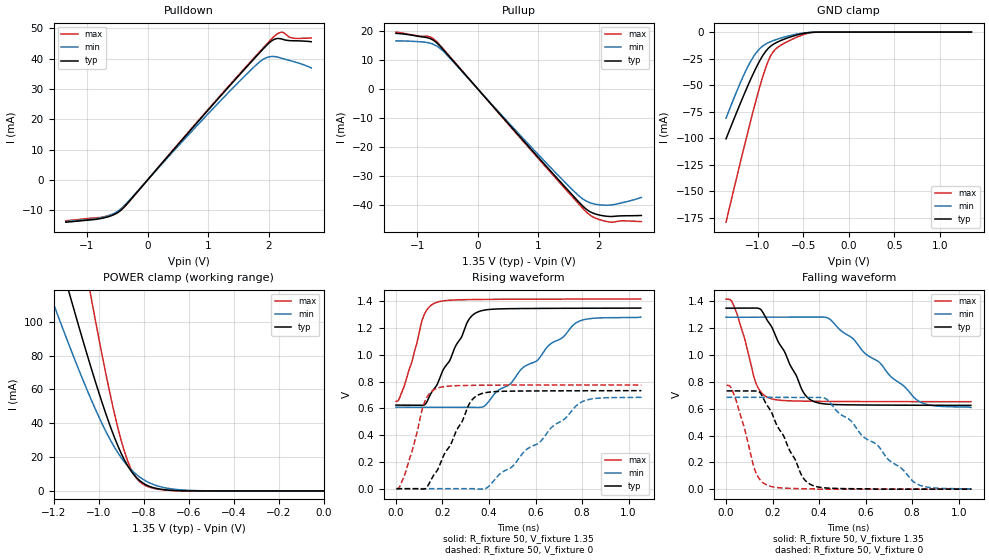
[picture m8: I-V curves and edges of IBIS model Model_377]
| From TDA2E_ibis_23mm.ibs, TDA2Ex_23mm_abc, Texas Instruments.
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| Model based on original model for DDR_SEIOPB_V
|   Sub model SR100_DRV40_1P35
[model]   Model_377
|[Description]  [1.35V-I/O-X-X]
|   , ,
|[Input Load]
|[Output Drive]
|Voltage   1.35V
|Mode   I/O
Model_type   I/O
Polarity   Non-Inverting
Enable   Active-Low
Vinl =  0.585
Vinh =  0.765
Cref =  15.0000pF
Rref =  100.0000M
Vref =  0V
Vmeas =  0.675
C_comp   2p   2p   2p
[Model Spec]
Vinl   0.585   0.55125   0.61875
Vinh   0.765   0.73125   0.79875
[Receiver Thresholds]
Tslew_ac = 5n
Vth= 0.675
Vth_max= 0.709
Vth_min= 0.608
Vinh_ac= 0.175
Vinh_dc= 0.1
Vinl_ac= -0.175
Vinl_dc= -0.1
[Temperature Range]   25   125   -40
[Voltage Range]   1.35   1.2825   1.4175
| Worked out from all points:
|   slope of the pulldown table from 0 to 0.203 V, typ, clamps not added: 43 ohm
|   slope of the pullup table from 0 to 0.203 V, typ, clamps not added: 42 ohm
|   GND clamp passes 1 mA (typ) near -0.48 V on its own axis
|   POWER clamp passes 1 mA (typ) near -0.72 V on its own axis
|   rising waveform, R_fixture 50, V_fixture 1.35: 20-80 % time 123ps typ, 279ps min, 71.1ps max; typ from 0.625 V to 1.35 V
|   rising waveform, R_fixture 50, V_fixture 0: 20-80 % time 122ps typ, 269ps min, 71.1ps max; typ from 0 V to 0.733 V
|   falling waveform, R_fixture 50, V_fixture 1.35: 20-80 % time 121ps typ, 254ps min, 71ps max; typ from 1.35 V to 0.625 V
|   falling waveform, R_fixture 50, V_fixture 0: 20-80 % time 122ps typ, 263ps min, 71ps max; typ from 0.733 V to 0 V
[POWER_clamp]
-1.35V    224.4mA    165.8mA    358.5mA
-1.214V   157mA      115.5mA    250.8mA
-1.132V   117.8mA    86.59mA    187.7mA
-1.118V   111.4mA    81.92mA    177.3mA
-1.036V   74.26mA    55.16mA    116.8mA
-954.5mV  40.7mA     31.91mA    61.06mA
-900mV    22.42mA    19.79mA    30.14mA
-859.1mV  12.48mA    13.09mA    13.96mA
-804.5mV  4.85mA     7.084mA    4.132mA
-736.4mV  1.313mA    2.9mA      1.073mA
-627.3mV  101.6uA    577.3uA    45.9uA
0V        75.63nA    322.4nA    418.5nA
[Pulldown]
-1.35V    -13.93mA   -13.71mA   -13.45mA
-736.4mV  -12.58mA   -12.32mA   -12.19mA
-531.8mV  -11.22mA   -10.8mA    -10.99mA
-409.1mV  -9.378mA   -8.926mA   -9.416mA
1.145V    26.32mA    24.88mA    26.57mA
1.718V    39.05mA    36.49mA    39.37mA
1.923V    43.49mA    39.91mA    43.83mA
2.005V    45.12mA    40.54mA    45.58mA
2.086V    46.28mA    40.65mA    47.24mA
2.209V    46.44mA    40.1mA     48.7mA
2.373V    45.86mA    39.19mA    46.8mA
2.7V      45.54mA    36.91mA    46.74mA
[Pullup]
-1.35V    19.14mA    16.53mA    19.57mA
-981.8mV  18.13mA    16.28mA    18.23mA
-818.2mV  17.57mA    15.91mA    18.13mA
-736.4mV  16.82mA    15.4mA     17.33mA
-613.6mV  14.56mA    13.83mA    14.83mA
1.064V    -25.08mA   -24.06mA   -25.52mA
1.555V    -36.41mA   -34.6mA    -37.03mA
1.759V    -40.9mA    -38.29mA   -41.73mA
1.923V    -42.98mA   -39.67mA   -44.36mA
2.127V    -43.9mA    -40.1mA    -45.7mA
2.291V    -43.85mA   -39.69mA   -45.73mA
2.7V      -43.64mA   -37.43mA   -45.74mA
[GND_clamp]
-1.35V    -100.7mA   -81.27mA   -179.3mA
-1.241V   -77.31mA   -57.61mA   -140mA
-1.132V   -54.83mA   -36.31mA   -101.6mA
-1.05V    -39.08mA   -23.36mA   -74mA
-968.2mV  -25.28mA   -14.71mA   -48.34mA
-913.6mV  -18.13mA   -11.32mA   -33.52mA
-859.1mV  -13.28mA   -9.024mA   -22.35mA
-831.8mV  -11.61mA   -8.091mA   -18.64mA
-777.3mV  -9.078mA   -6.444mA   -14.07mA
-531.8mV  -1.871mA   -1.307mA   -3.441mA
-368.2mV  -88.76uA   -111.2uA   -158uA
1.35V     75.63nA    385.5nA    349.4nA
[Ramp]
dV/dt_f 0.43564356/0.12167506n  0.4048292/0.25520489n 0.45934649/71.063488p
dV/dt_r 0.44154169/0.12285168n 0.41311001/0.27207171n 0.46695742/71.285994p
R_load = 50
[Rising Waveform]
R_fixture = 50
V_fixture = 1.35
V_fixture_min = 1.2825
V_fixture_max = 1.4175
0s        624.9mV    609.4mV    653.3mV
36.58ps   624.2mV    609.3mV    770.4mV
118.4ps   624.2mV    609.3mV    1.288V
169ps     756.2mV    609.4mV    1.389V
310.2ps   1.255V     609mV      1.413V
353.6ps   1.322V     607.2mV    1.414V
490ps     1.346V     780.7mV    1.416V
542ps     1.347V     898.4mV    1.417V
780.1ps   1.349V     1.245V     1.417V
1.053ns   1.35V      1.282V     1.417V
[Rising Waveform]
R_fixture = 50
V_fixture = 0
V_fixture_min = 0
V_fixture_max = 0
2.392ps   0V         0V         0V
39.37ps   0V         0V         112.5mV
122.3ps   -2.174mV   0V         643.5mV
172.6ps   124.2mV    0V         747.4mV
315.5ps   634.4mV    0V         772.3mV
360.4ps   705.7mV    -3.445mV   773.2mV
499ps     729.3mV    163.5mV    774.7mV
555.3ps   730.3mV    283.5mV    775mV
793.2ps   732.1mV    643.5mV    775.5mV
1.055ns   733mV      684.9mV    775.7mV
[Falling Waveform]
R_fixture = 50
V_fixture = 1.35
V_fixture_min = 1.2825
V_fixture_max = 1.4175
0s        1.35V      1.282V     1.417V
22.83ps   1.35V      1.283V     1.405V
45.37ps   1.35V      1.283V     1.315V
131.2ps   1.351V     1.283V     779.7mV
180.5ps   1.251V     1.283V     682.8mV
330.8ps   727.2mV    1.282V     656.5mV
377.9ps   653.2mV    1.283V     655.4mV
447.3ps   632.6mV    1.266V     654.3mV
830.9ps   625.9mV    653.5mV    652.6mV
1.053ns   624.9mV    609.4mV    652.5mV
[Falling Waveform]
R_fixture = 50
V_fixture = 0
V_fixture_min = 0
V_fixture_max = 0
2.392ps   733mV      684.9mV    774.8mV
21.01ps   733.2mV    685mV      758.5mV
43.12ps   733.2mV    685mV      662.3mV
126.2ps   733.2mV    685mV      132.4mV
176.8ps   625mV      685mV      29.73mV
325.6ps   101mV      684.8mV    3.469mV
369.9ps   29.39mV    685.2mV    2.346mV
436.6ps   8.078mV    665.8mV    0V
817.5ps   0V         41.74mV    0V
1.055ns   0V         0V         0V
